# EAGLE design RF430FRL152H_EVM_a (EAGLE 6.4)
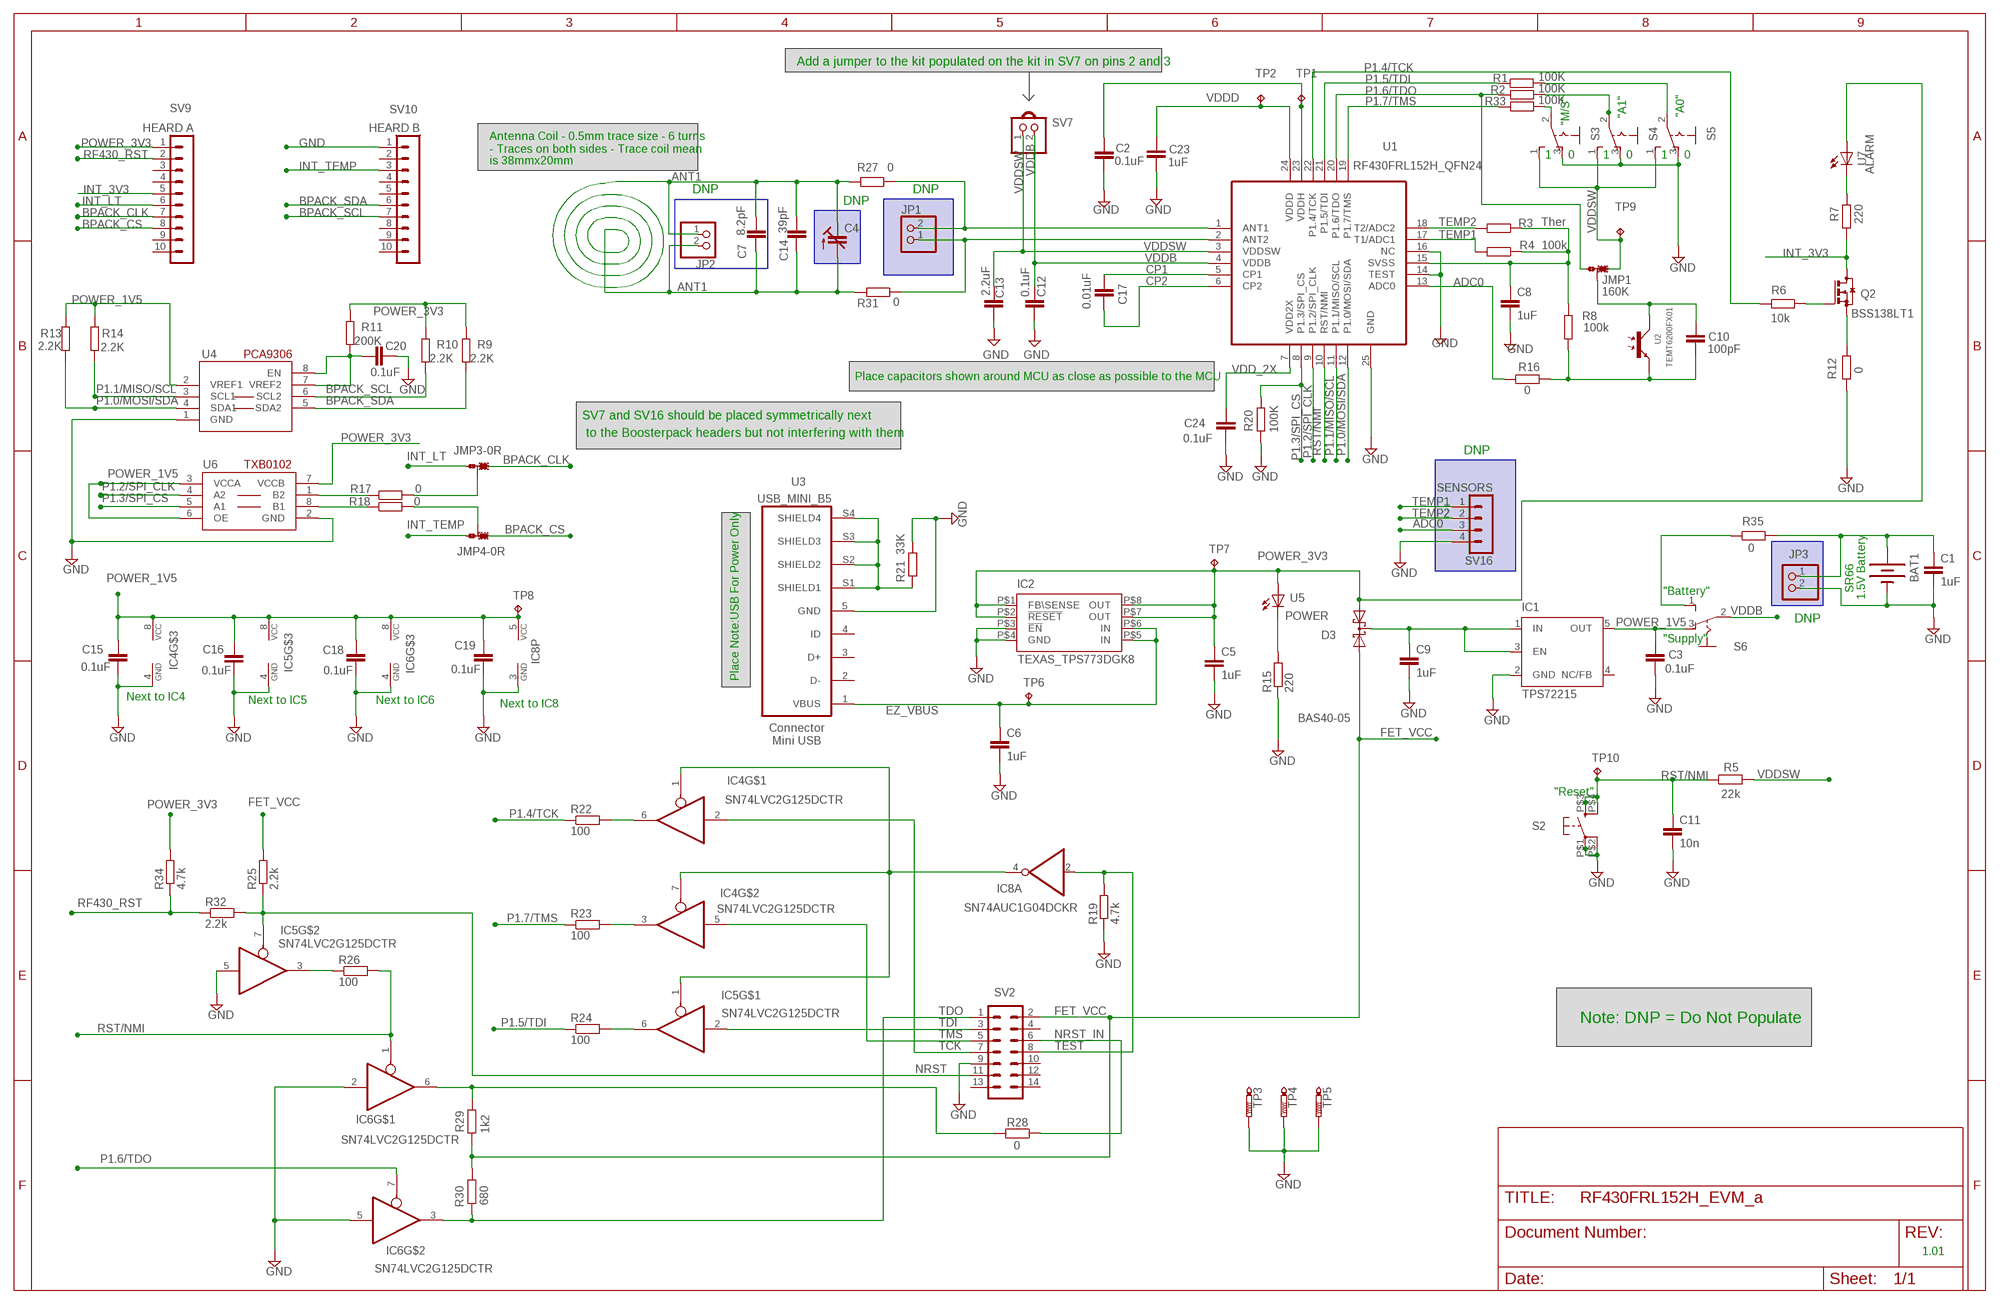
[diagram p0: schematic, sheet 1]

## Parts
BAT1  SPARKFUN_BATTERY12MM  [SPARKFUN_BATTCON_12MM]
C1  1uF  LAUNCHPAD_CAP0603  [ROY_CAP_0603]
C2  0.1uF  LAUNCHPAD_CAP0603  [ROY_CAP_0603]
C3  0.1uF  LAUNCHPAD_CAP0603  [ROY_CAP_0603]
C4  C-TRIMM_C-TRIMM3008  [C-TRIMM_3008]
C5  1uF  LAUNCHPAD_CAP0603  [ROY_CAP_0603]
C6  1uF  LAUNCHPAD_CAP0603  [ROY_CAP_0603]
C7  8.2pF  LAUNCHPAD_CAP0603  [ROY_CAP_0603]
C8  1uF  LAUNCHPAD_CAP0603  [ROY_CAP_0603]
C9  1uF  LAUNCHPAD_CAP0603  [ROY_CAP_0603]
C10  100pF  LAUNCHPAD_CAP0603  [ROY_CAP_0603]
C11  10n  LAUNCHPAD_CAP0603  [ROY_CAP_0603]
C12  0.1uF  LAUNCHPAD_CAP0603  [ROY_CAP_0603]
C13  2.2uF  LAUNCHPAD_CAP0603  [ROY_CAP_0603]
C14  39pF  LAUNCHPAD_CAP0603  [ROY_CAP_0603]
C15  0.1uF  LAUNCHPAD_CAP0603  [ROY_CAP_0603]
C16  0.1uF  LAUNCHPAD_CAP0603  [ROY_CAP_0603]
C17  0.01uF  LAUNCHPAD_CAP0603  [ROY_CAP_0603]
C18  0.1uF  LAUNCHPAD_CAP0603  [ROY_CAP_0603]
C19  0.1uF  LAUNCHPAD_CAP0603  [ROY_CAP_0603]
C20  0.1uF  LAUNCHPAD_CAP0603  [ROY_CAP_0603]
C23  1uF  LAUNCHPAD_CAP0603  [ROY_CAP_0603]
C24  0.1uF  LAUNCHPAD_CAP0603  [ROY_CAP_0603]
D3  BAS40-05  [SOT23]
IC1  TPS72215  TEXAS_TPS77015  [TEXAS_SOT23-DBV]
IC2  TEXAS_TPS773DGK8  [DGK]
IC4  SN74LVC2G125DCTR  APOLLO_74LVC2G125DCT  [APOLLO_SSOP08]
IC5  SN74LVC2G125DCTR  APOLLO_74LVC2G125DCT  [APOLLO_SSOP08]
IC6  SN74LVC2G125DCTR  APOLLO_74LVC2G125DCT  [APOLLO_SSOP08]
IC8  SN74AUC1G04DCKR  74XX-LITTLE-DE_74AUC1G04DCK  [74XX-LITTLE-DE_SC70-5]
JMP1  160K-JUMPB  0R-JUMPB  [B0R-JMP]
JMP3  0R-JUMPB  [B0R-JMP]
JMP4  0R-JUMPB  [B0R-JMP]
JP1  APOLLO_PINHD-1X2  [APOLLO_1X02]
JP2  APOLLO_PINHD-1X2  [APOLLO_1X02]
JP3  APOLLO_PINHD-1X2  [APOLLO_1X02]
Q2  BSS138LT1  BSS123  [SOT23]
R1  100K  LAUNCHPAD_RES0603  [ROY_RES_0603]
R2  100K  LAUNCHPAD_RES0603  [ROY_RES_0603]
R3  Ther  LAUNCHPAD_RES0603  [ROY_RES_0603]
R4  100k  LAUNCHPAD_RES0603  [ROY_RES_0603]
R5  22k  LAUNCHPAD_RES0603  [ROY_RES_0603]
R6  10k  LAUNCHPAD_RES0603  [ROY_RES_0603]
R7  220  LAUNCHPAD_RES0603  [ROY_RES_0603]
R8  100k  LAUNCHPAD_RES0603  [ROY_RES_0603]
R9  2.2K  LAUNCHPAD_RES0603  [ROY_RES_0603]
R10  2.2K  LAUNCHPAD_RES0603  [ROY_RES_0603]
R11  200K  LAUNCHPAD_RES0603  [ROY_RES_0603]
R12  0  LAUNCHPAD_RES0603  [ROY_RES_0603]
R13  2.2K  LAUNCHPAD_RES0603  [ROY_RES_0603]
R14  2.2K  LAUNCHPAD_RES0603  [ROY_RES_0603]
R15  220  LAUNCHPAD_RES0603  [ROY_RES_0603]
R16  0  LAUNCHPAD_RES0603  [ROY_RES_0603]
R17  0  LAUNCHPAD_RES0603  [ROY_RES_0603]
R18  0  LAUNCHPAD_RES0603  [ROY_RES_0603]
R19  4.7k  LAUNCHPAD_RES0603  [ROY_RES_0603]
R20  100K  LAUNCHPAD_RES0603  [ROY_RES_0603]
R21  33K  LAUNCHPAD_RES0603  [ROY_RES_0603]
R22  100  LAUNCHPAD_RES0603  [ROY_RES_0603]
R23  100  LAUNCHPAD_RES0603  [ROY_RES_0603]
R24  100  LAUNCHPAD_RES0603  [ROY_RES_0603]
R25  2.2k  LAUNCHPAD_RES0603  [ROY_RES_0603]
R26  100  LAUNCHPAD_RES0603  [ROY_RES_0603]
R27  0  LAUNCHPAD_RES0603  [ROY_RES_0603]
R28  0  LAUNCHPAD_RES0603  [ROY_RES_0603]
R29  1k2  LAUNCHPAD_RES0603  [ROY_RES_0603]
R30  680  LAUNCHPAD_RES0603  [ROY_RES_0603]
R31  0  LAUNCHPAD_RES0603  [ROY_RES_0603]
R32  2.2k  LAUNCHPAD_RES0603  [ROY_RES_0603]
R33  100K  LAUNCHPAD_RES0603  [ROY_RES_0603]
R34  4.7k  LAUNCHPAD_RES0603  [ROY_RES_0603]
R35  0  LAUNCHPAD_RES0603  [ROY_RES_0603]
S2  HERCULES_LAUNCHPAD_V1.1_LAUNCHPAD_T062ST06B-025FWT01B  [SW-6.1*3.7]
S3  M251  [M251]
S4  M251  [M251]
S5  M251  [M251]
S6  M251  [M251]
SV2  ML14  [ML14]
SV7  APOLLO_PINHD-1X2  [APOLLO_1X02]
SV9  HEARD A  CON-LSTB_MA10-1W  [CON-LSTB_MA10-1W]
SV10  HEARD B  CON-LSTB_MA10-1W  [CON-LSTB_MA10-1W]
SV16  SENSORS  MA04-1  [MA04-1]
TP1  TPB1,27  [B1,27]
TP2  TPB1,27  [B1,27]
TP3  PTR1PAD1-13  [P1-13]
TP4  PTR1PAD1-13  [P1-13]
TP5  PTR1PAD1-13  [P1-13]
TP6  TPB1,27  [B1,27]
TP7  TPB1,27  [B1,27]
TP8  TPB1,27  [B1,27]
TP9  TPB1,27  [B1,27]
TP10  TPB1,27  [B1,27]
U1  RF430FRL152H_QFN24  APOLLO_APOLLO_24PINQFN24  [QFN24]
U2  TEMT6200FX01  LAUNCHPAD_TEMT60006200  [LAUNCHPAD_0805]
U3  USB_MINI_B5  [USB_MINI_B]
U4  SPARKFUN_PCA9306DCU  [MY_DCU_R-PDSO-G8]
U5  POWER  LEDCHIP-LED0603  [CHIP-LED0603]
U6  TXB0102  [DCU_R-PDSO-G8]
U7  ALARM  LEDCHIP-LED0603  [CHIP-LED0603]
U$1  ROY_JUMPER  [ROY_JUMPER]

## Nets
ADC0: R16.1 SV16.3 U1.13(ADC0)
ANT1: C4.+(E) C4.-(A) C7.1 C7.2 C14.1 C14.2 JP2.1 JP2.2 R27.2 R31.2
BPACK_CLK: JMP3.1 SV9.7
BPACK_CLK_N: JMP3.2 R17.2
BPACK_CS: JMP4.3 SV9.8
BPACK_CS_N: JMP4.2 R18.2
BPACK_SCL: R10.2 SV10.7 U4.6(SCL2)
BPACK_SDA: R9.2 SV10.6 U4.5(SDA2)
CP1: C17.2 U1.5(CP1)
CP2: C17.1 U1.6(CP2)
EZ_VBUS: C6.1 IC2.P$5(IN) IC2.P$6(IN) TP6.TP U3.1(VBUS)
FET_VCC: D3.2(A2) R25.2 R29.1 R30.1 SV2.2
GND: BAT1.GND(-) C1.2 C2.2 C3.1 C5.2 C6.2 C8.2 C9.2 C11.2 C12.1 C13.1 C15.1 C16.1 C18.1 C19.1 C20.1 C23.2 C24.1 IC1.2(GND) IC2.P$3(!EN) IC2.P$4(GND) IC4.4(GND) IC5.4(GND) IC5.5(I) IC6.2(I) IC6.4(GND) IC6.5(I) IC8.3(P:GND) JP3.2 R12.1 R15.1 R19.1 R20.1 R21.2 S2.P$1 S2.P$2 S3.3(S) S4.3(S) S5.3(S) SV2.9 SV10.1 SV16.4 TP3.TP TP4.TP TP5.TP U1.14(TEST) U1.16(NC) U1.25(GND) U3.5(GND) U4.1(GND) U6.2(GND)
INT_3V3: Q2.3(D) R7.1 SV9.5
INT_LT: JMP3.3 SV9.6
INT_TEMP: JMP4.1 SV10.3
N$1: C9.1 D3.3(C) IC1.1(IN) IC1.3(EN)
N$2: C10.1 R8.2 R16.2 U2.2(E)
N$4: JP1.2 R27.1 U1.1(ANT1)
N$5: C8.1 R3.1 R4.1 R8.1 U1.15(SVSS)
N$6: JP1.1 R31.1 U1.2(ANT2)
N$7: R7.2 U7.C
N$8: R35.1 S6.1(O)
N$9: C20.2 R11.2 U4.7(VREF2) U4.8(EN)
N$10: R15.2 U5.C
N$12: Q2.2(S) R12.2
N$13: Q2.1(G) R6.1
N$14: BAT1.PWR@1(+) C1.1 JP3.1 R35.2
N$15: R1.2 S5.2(P)
N$17: R17.1 U6.1(B2)
N$18: R18.1 U6.8(B1)
N$21: C10.2 JMP1.2 U2.1(C)
N$22: R21.1 U3.S1(SHIELD1) U3.S2(SHIELD2) U3.S3(SHIELD3) U3.S4(SHIELD4)
N$23: IC4.1(OE) IC4.7(OE) IC5.1(OE) IC8.4(A:O)
N$24: IC4.6(O) R22.2
N$25: IC4.3(O) R23.2
N$26: IC5.6(O) R24.2
N$27: R2.1 S4.2(P)
N$28: IC5.3(O) R26.1
N$29: R33.1 S3.2(P)
N$30: IC6.6(O) R28.2 R29.2
NRST: IC5.7(OE) R25.1 R32.2 SV2.11
NRST_IN: R28.1 SV2.6
P1.0/MOSI/SDA: R13.2 U1.12(P1.0/MOSI/SDA) U4.4(SDA1)
P1.1/MISO/SCL: R14.2 U1.11(P1.1/MISO/SCL) U4.3(SCL1)
P1.2/SPI_CLK: U1.9(P1.2/SPI_CLK) U6.4(A2)
P1.3/SPI_CS: R20.2 U1.8(P1.3/SPI_CS) U6.5(A1)
P1.4/TCK: R6.2 R22.1 U1.22(P1.4/TCK)
P1.5/TDI: R1.1 R24.1 U1.21(P1.5/TDI)
P1.6/TDO: IC6.7(OE) JMP1.3 R2.2 U1.20(P1.6/TDO)
P1.7/TMS: R23.1 R33.2 U1.19(P1.7/TMS)
POWER_1V5: C3.2 C15.2 C16.2 C18.2 C19.2 IC1.5(OUT) IC4.8(VCC) IC5.8(VCC) IC6.8(VCC) IC8.5(P:VCC) R13.1 R14.1 S6.3(S) TP8.TP U4.2(VREF1) U6.3(VCCA) U6.6(OE)
POWER_3V3: C5.1 D3.1(A1) IC2.P$1(FB\SENSE) IC2.P$2(!RESET) IC2.P$7(OUT) IC2.P$8(OUT) R9.1 R10.1 R11.1 R34.2 SV9.1 TP7.TP U5.A U6.7(VCCB) U7.A
RF430_RST: R32.1 R34.1 SV9.2
RST/NMI: C11.1 IC6.1(OE) R5.1 R26.2 S2.P$3 S2.P$4 TP10.TP U1.10(RST/NMI)
TCK: IC4.2(I) SV2.7
TDI: IC5.2(I) SV2.3
TDO: IC6.3(O) R30.2 SV2.1
TEMP1: R4.2 SV16.1 U1.17(T1/ADC1)
TEMP2: R3.2 SV16.2 U1.18(T2/ADC2)
TEST: IC8.2(A:I) R19.2 SV2.8
TMS: IC4.5(I) SV2.5
VDD_2X: C24.2 U1.7(VDD2X)
VDDB: C12.2 S6.2(P) SV7.2 U1.4(VDDB)
VDDD: C23.1 TP2.TP U1.24(VDDD)
VDDH: C2.1 TP1.TP U1.23(VDDH)
VDDSW: C13.2 JMP1.1 R5.2 S3.1(O) S4.1(O) S5.1(O) SV7.1 TP9.TP U1.3(VDDSW)
Unconnected: IC1.4(NC/FB) SV2.4 SV2.10 SV2.12 SV2.13 SV2.14 SV9.3 SV9.4 SV9.9 SV9.10 SV10.2 SV10.4 SV10.5 SV10.8 SV10.9 SV10.10 U3.2(D-) U3.3(D+)

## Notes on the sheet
- Add a jumper to the kit populated on the kit in SV7 on pins 2 and 3
- "M/S" | "A1" | "A0"
- Pickup coil
- Antenna Coil - 0.5mm trace size - 6 turns
- - Traces on both sides - Trace coil mean
- 1 | 0 | 1 | 0 | 1 | 0
- is 38mmx20mm
- DNP | DNP
- DNP
- JMP1
- 160K
- Place capacitors shown around MCU as close as possible to the MCU
- SV7 and SV16 should be placed symmetrically next
- to the Boosterpack headers but not interfering with them
- DNP
- "Battery" | SR66
- 1.5V Battery
- DNP
- "Supply"
- Place Note:USB For Power Only
- Next to IC4
- Next to IC5 | Next to IC6
- Next to IC8
- Connector
- Mini USB
- "Reset"
- Note: DNP = Do Not Populate
- 1.01

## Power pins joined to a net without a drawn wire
ID: U3.4(ID)

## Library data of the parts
BAT1 = RF430FRL152H_EVM_a:SPARKFUN_BATTERY: Battery Holders
C1-C3 C5-C20 C23 C24 = roy:LAUNCHPAD_CAP
C4 = RF430FRL152H_EVM:C-TRIMM_C-TRIMM: Trimm capacitor; OC_FARNELL: unknown; OC_NEWARK: unknown
D3 = diode:BAS40-05: Silicon Schottky Diodes General-purpose diode for high-speed switching
IC1 = RF430FRL152H_EVM_a:TEXAS_TPS770*: ULTRALOW-POWER 50-mA LOW-DROPOUT LINEAR REGULATORS 50-mA Low-Dropout Regulator Source: http://focus.ti.com/lit/ds/symlink/tps77001.pdf; MF: TEXAS INSTRUMENT CONNECTORS; MPN: TPS77015DBVT; OC_FARNELL: 1412879; OC_NEWARK: 77C1175
IC2 = RF430FRL152H_EVM_a:TEXAS_TPS773*: 250-mA LDO REGULATORS WITH RESET OUTPUT WITH 8-PIN MSOP PACKAGING Source: http://focus.ti.com/lit/ds/symlink/tps77333.pdf
IC4-IC6 = RF430FRL152H_EVM_a:APOLLO_74*2G125: Dual line drivers with 3-state outputs.
IC8 = RF430FRL152H_EVM_a:74XX-LITTLE-DE_74*1G04: INVERTER Gate
JMP1 JMP3 JMP4 = jump-0r-smd:0R-JUMP: SMD 0R 0805 Jumper
JP1-JP3 SV7 = RF430FRL152H_EVM:APOLLO_PINHD-1X2: PIN HEADER
Q2 = transistor-small-signal:BSS123: N-CHANNEL MOS FET
R1-R35 = roy:LAUNCHPAD_RES
S2 = yw8:HERCULES_LAUNCHPAD_V1.1_LAUNCHPAD_T062S
S3-S6 = switch:M251: SLIDING SWITCH Mors, distributor Buerklin, 11G702
SV2 = con-ml:ML14: HARTING; OC_FARNELL: unknown; OC_NEWARK: unknown
SV9 SV10 = RF430FRL152H_EVM_a:CON-LSTB_MA10-1W: PIN HEADER; OC_FARNELL: unknown; OC_NEWARK: unknown
SV16 = con-lstb:MA04-1: PIN HEADER; OC_FARNELL: unknown; OC_NEWARK: unknown
TP1 TP2 TP6-TP10 = testpad:TP: Test pad
TP3-TP5 = testpad:PTR1: TEST PIN
U1 = RF430FRL152H_EVM_a:APOLLO_APOLLO_24PIN
U2 = roy:LAUNCHPAD_TEMT6000
U3 = susbfet:USB_MINI_B5
U4 = RF430FRL152H_EVM_a:SPARKFUN_PCA9306
U5 U7 = led:LED: LED
U6 = My:TXB0102
U$1 = roy:ROY_JUMPER

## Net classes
1 Ground: width 0.203 mm, drill 0.61 mm

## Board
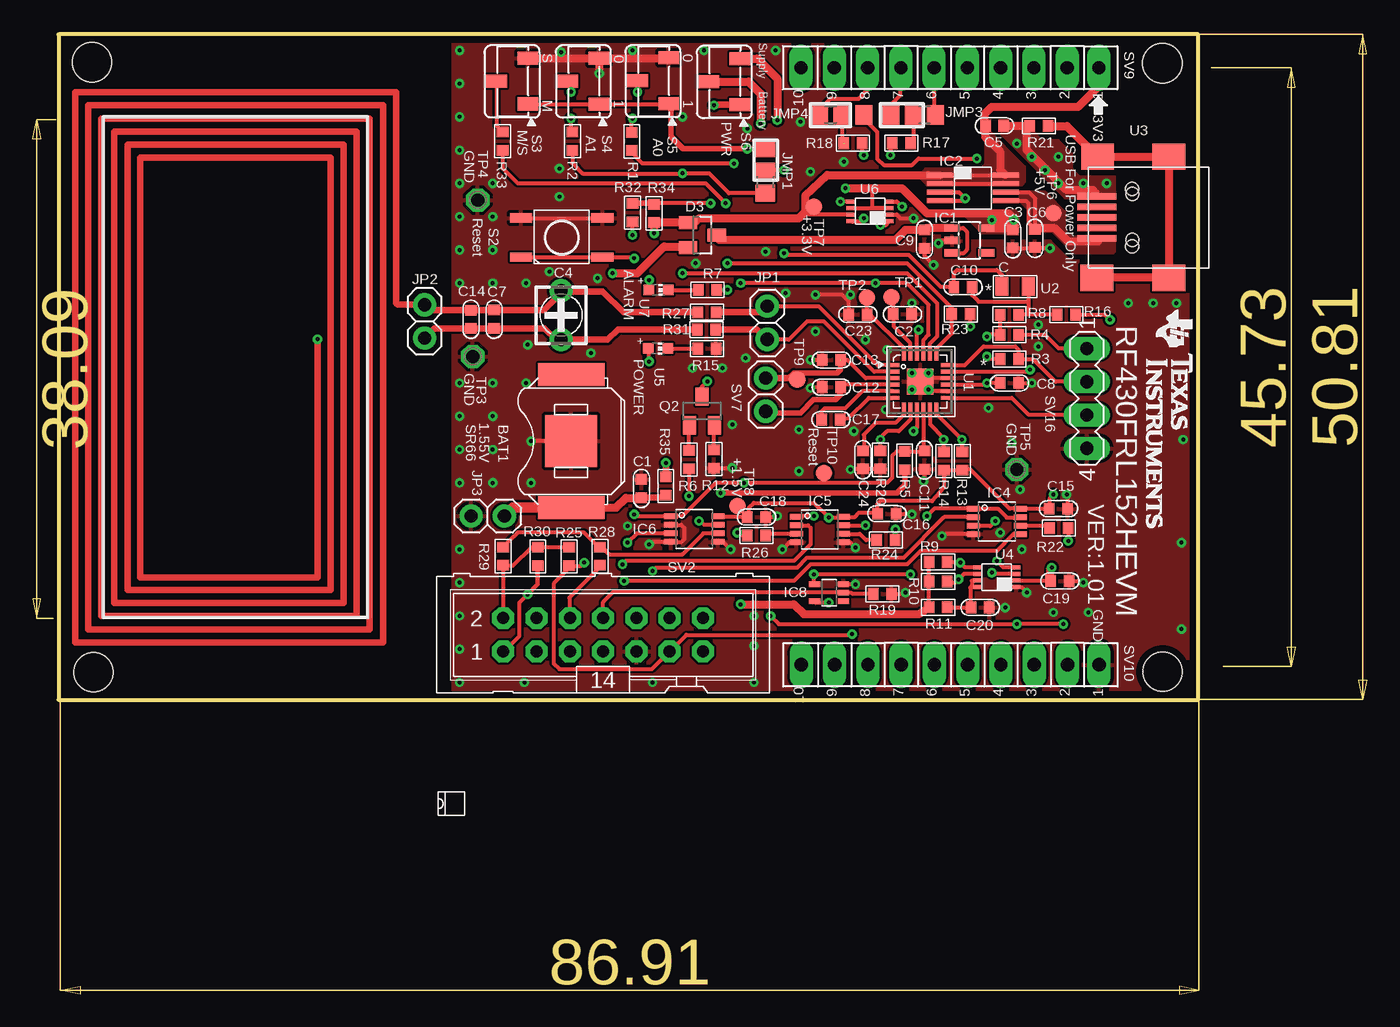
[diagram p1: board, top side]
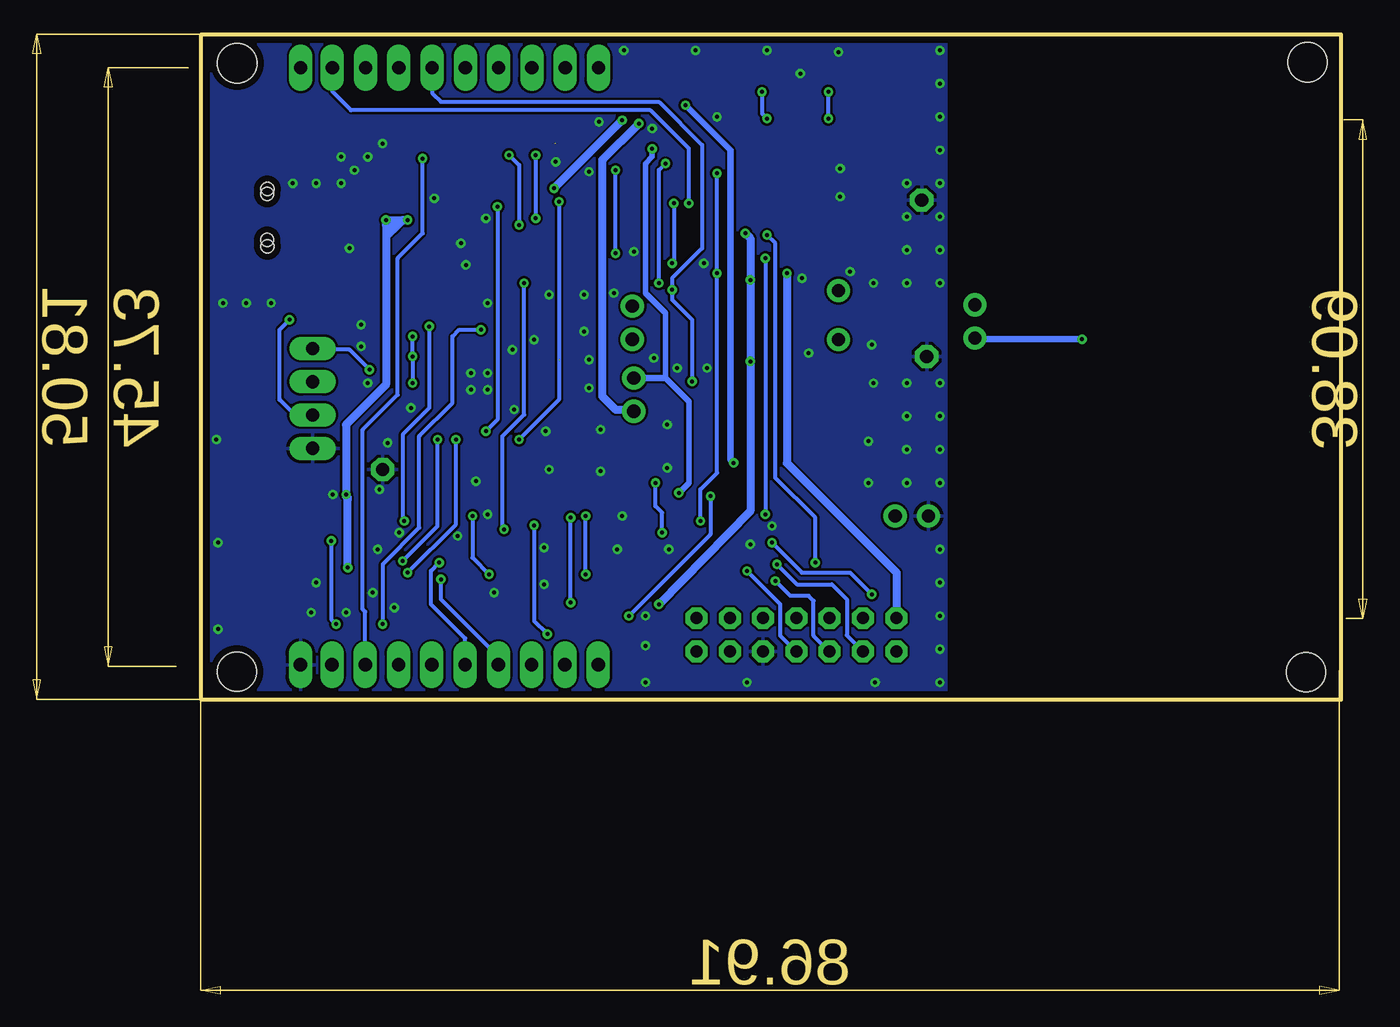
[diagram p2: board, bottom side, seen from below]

Size 101.84 x 73.3 mm. Coordinates in mm from the lower left corner, seen from the top.
Outline: 1.98,22.47 88.98,22.47 88.98,73.28 1.98,73.28 1.98,22.47
Copper layers (1*16): Top 0.035mm / dielectric 1.5mm / Bottom 0.035mm
Design rules "default": minimum track width 8mil, minimum drill 10mil, track to track 7mil, track to pad 7mil, pad to pad 7mil, via to via 7mil, smd to smd 0mil, copper to edge 20mil, drill to drill 10mil, minimum pad ring 15mil, minimum via ring 8mil, stop-mask expansion 4mil, vias tented up to drill 0mil, thermal gap 10mil
Holes 3 mm at 4.52,71.15 4.65,24.57 86.25,24.61 86.24,71.07
Holes 1 mm at 83.95,61.09 83.95,57.58

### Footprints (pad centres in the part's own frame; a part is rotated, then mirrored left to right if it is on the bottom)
SPARKFUN_BATTCON_12MM = smd 3.962 x 3.962: GND 0,0 | smd 1.778 x 5.08: PWR@1 -5.08,0; PWR@2 5.08,0
ROY_CAP_0603 = smd 0.8 x 0.9: 1 -0.7,0; 2 0.7,0
C-TRIMM_3008 = drill 1: + -1.875,0; - 1.875,0
SOT23 = smd 1 x 1.4: 1 -0.95,-1.1; 2 0.95,-1.1; 3 0,1.1
TEXAS_SOT23-DBV = smd 0.55 x 1.2: 1 -0.95,-1.3; 2 0,-1.3; 3 0.95,-1.3; 4 0.95,1.3; 5 -0.95,1.3
DGK = smd 0.4 x 2: P$1 0,0; P$2 0.65,0; P$3 1.3,0; P$4 1.95,0; P$5 1.95,5.05; P$6 1.3,5.05; P$7 0.65,5.05; P$8 0,5.05
APOLLO_SSOP08 = smd 0.4 x 1: 1 -0.975,-1.8; 2 -0.325,-1.8; 3 0.325,-1.8; 4 0.975,-1.8; 5 0.975,1.8; 6 0.325,1.8; 7 -0.325,1.8; 8 -0.975,1.8
74XX-LITTLE-DE_SC70-5 = smd 0.4 x 0.85: 1 -0.65,-1.1; 2 0,-1.1; 3 0.65,-1.1; 4 0.65,1.1; 5 -0.65,1.1
B0R-JMP = smd 1.5 x 1.3: 1 0,1.7; 2 0,0; 3 0,-1.7
APOLLO_1X02 = drill 1.016: 1 -1.27,0; 2 1.27,0
ROY_RES_0603 = smd 0.8 x 0.9: 1 -0.7,0; 2 0.7,0
SW-6.1*3.7 = smd 1.7 x 0.7: P$1 -3.1,1.5; P$2 3.1,1.5; P$3 -3.1,-1.5; P$4 3.1,-1.5
M251 = smd 1 x 1.6: 1 -1.75,-1.2; 2 0,1.2; 3 1.75,-1.2
ML14 = drill 0.914 octagon: 1 -7.62,-1.27; 2 -7.62,1.27; 3 -5.08,-1.27; 4 -5.08,1.27; 5 -2.54,-1.27; 6 -2.54,1.27; 7 0,-1.27; 8 0,1.27; 9 2.54,-1.27; 10 2.54,1.27; 11 5.08,-1.27; 12 5.08,1.27; 13 7.62,-1.27; 14 7.62,1.27
CON-LSTB_MA10-1W = drill 1.016 long: 1 -11.303,0; 2 -8.89,0; 3 -6.35,0; 4 -3.81,0; 5 -1.27,0; 6 1.27,0; 7 3.81,0; 8 6.35,0; 9 8.89,0; 10 11.43,0
MA04-1 = drill 1.016 long: 1 -3.81,0; 2 -1.27,0; 3 1.27,0; 4 3.81,0
B1,27 = smd 1.27 x 1.27: TP 0,0
P1-13 = drill 1 pad 1.676 octagon: TP 0,0
QFN24 = smd 1 x 0.3: 1 -2.1,1.25; 2 -2.1,0.75; 3 -2.1,0.25; 4 -2.1,-0.25; 5 -2.1,-0.75; 6 -2.1,-1.25; 13 2.1,-1.25; 14 2.1,-0.75; 15 2.1,-0.25; 16 2.1,0.25; 17 2.1,0.75; 18 2.1,1.25 | smd 0.3 x 1: 7 -1.25,-2.1; 8 -0.75,-2.1; 9 -0.25,-2.1; 10 0.25,-2.1; 11 0.75,-2.1; 12 1.25,-2.1; 19 1.25,2.1; 20 0.75,2.1; 21 0.25,2.1; 22 -0.25,2.1; 23 -0.75,2.1; 24 -1.25,2.1 | smd 2 x 2: 25 0,0
LAUNCHPAD_0805 = smd 1 x 1.4: 1 -1,0; 2 1,0
USB_MINI_B = smd 0.5 x 3: 1 -1.6,8.55; 2 -0.8,8.55; 3 0,8.55; 4 0.8,8.55; 5 1.6,8.55 | smd 2 x 2.5: S1 -4.6,8.55; S2 -4.6,3.05; S3 4.65,3.05; S4 4.65,8.5 | hole 1.016: -2.2,5.85; 2.2,5.85
MY_DCU_R-PDSO-G8 = smd 0.3 x 0.6: 1 -0.75,-1.5; 2 -0.25,-1.5; 3 0.25,-1.5; 4 0.75,-1.5; 5 0.75,1.5; 6 0.25,1.5; 7 -0.25,1.5; 8 -0.75,1.5
CHIP-LED0603 = smd 0.8 x 0.8: A 0,-0.75; C 0,0.75
DCU_R-PDSO-G8 = smd 0.3 x 0.6: 1 -0.75,-1.5; 2 -0.25,-1.5; 3 0.25,-1.5; 4 0.75,-1.5; 5 0.75,1.5; 6 0.25,1.5; 7 -0.25,1.5; 8 -0.75,1.5

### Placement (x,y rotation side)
BAT1  41.1,42.22 90 top
C1  46.46,38.6 90 top
C2  66.4,51.91 0 top
C3  74.81,57.66 90 top
C4  40.33,51.83 270 top
C5  73.43,66.31 0 top
C6  76.5,57.7 270 top
C7  35.22,51.52 90 top
C8  74.56,46.67 0 top
C9  68.09,57.63 270 top
C10  71.02,53.98 180 top
C11  68.09,40.77 270 top
C12  60.97,46.34 0 top
C13  60.97,48.42 0 top
C14  33.45,51.52 90 top
C15  78.31,37.05 180 top
C16  65.22,36.67 180 top
C17  60.94,43.86 180 top
C18  55.26,36.41 180 top
C19  78.42,31.53 180 top
C20  72.33,29.51 180 top
C23  62.99,51.89 180 top
C24  63.37,40.79 90 top
D3  51.12,57.95 270 top
IC1  71.5,57.54 270 top
IC2  69.25,62.52 270 top
IC4  73.61,36.08 270 top
IC5  60.09,35.46 270 top
IC6  50.51,35.5 270 top
IC8  60.8,30.65 90 top
JMP1  55.93,62.83 0 top
JMP3  67.23,67.12 90 top
JMP4  61.76,67.13 270 top
JP1  56.07,51.25 90 top
JP2  29.91,51.35 270 top
JP3  34.74,36.5 180 top
Q2  51.09,44.52 0 top
R1  45.73,65.1 90 top
R2  41.2,65.12 270 top
R3  74.56,48.49 0 top
R4  74.55,50.34 0 top
R5  66.57,40.73 270 top
R6  50.11,40.8 270 top
R7  51.51,53.76 180 top
R8  74.55,51.86 0 top
R9  69.13,32.99 0 top
R10  69.13,31.51 0 top
R11  69.13,29.53 0 top
R12  52,40.85 90 top
R13  70.97,40.69 90 top
R14  69.57,40.69 90 top
R15  51.48,49.29 180 top
R16  78.91,51.88 180 top
R17  66.31,64.96 0 top
R18  62.62,64.97 180 top
R19  64.87,30.55 180 top
R20  64.72,40.8 90 top
R21  76.8,66.28 180 top
R22  78.35,35.57 180 top
R23  70.86,51.91 0 top
R24  65.13,34.67 180 top
R25  40.94,33.4 90 top
R26  55.25,35.02 180 top
R27  51.48,52.06 180 top
R28  43.3,33.43 90 top
R29  35.9,33.43 90 top
R30  38.56,33.41 270 top
R31  51.43,50.74 180 top
R32  45.78,59.67 270 top
R33  35.87,65.12 270 top
R34  47.44,59.61 270 top
R35  48.33,38.78 270 top
S2  40.38,57.76 0 top
S3  36.6,69.71 90 top
S4  42.04,69.71 90 top
S5  47.35,69.73 90 top
S6  52.79,69.67 90 top
SV2  43.54,27.43 0 top
SV7  55.95,45.77 270 top
SV9  70.08,70.73 180 top
SV10  70.1,25.14 180 top
SV16  80.48,45.48 270 top
TP1  65.55,53.22 0 top
TP2  63.68,53.19 0 top
TP3  33.6,48.69 0 top
TP4  33.98,60.62 0 top
TP5  75.13,40.05 0 top
TP6  77.92,59.61 0 top
TP7  59.63,60.12 0 top
TP8  53.79,37.26 0 top
TP9  58.36,46.91 0 top
TP10  60.39,39.8 0 top
U1  67.75,46.77 0 top
U2  75,54.02 0 top
U3  89.79,59.29 90 top
U4  73.6,31.82 90 top
U5  47.74,49.29 270 top
U6  63.92,59.77 90 top
U7  47.78,53.76 270 top
U$1  32.99,13.65 90 top
U$4  [LOGO16_TPLACE]  84.83,52.34 270 top

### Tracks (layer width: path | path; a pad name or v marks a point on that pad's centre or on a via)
ADC0  (via drill 0.3)
  Top 0.305: SV16.3 76.05,44.21 74.73,45.52 U1.13 | R16.1 81.84,51.88 v82.24,51.48
  Bottom 0.305: SV16.3 81.82,44.21 83,45.39 83,50.72 v82.24,51.48
ANT1  (via drill 0.3)
  Top 0.5: v21.73,50 21.73,31.82 8.21,31.82 8.21,63.85 22.73,63.85 22.73,30.85 7.23,30.85 7.23,64.85 23.73,64.85 23.73,29.85 6.23,29.85 6.23,65.85 24.73,65.85 24.73,28.85 5.23,28.85 5.23,66.85 25.73,66.85 25.73,27.85 4.23,27.85 4.23,67.85 26.73,67.85 26.73,26.85 3.23,26.85 3.23,68.85 27.73,68.85 27.73,52.77 27.88,52.62 JP2.1 30.45,52.22 C14.2 38.39,52.22 C7.2 39.04,52.22 40.46,53.64 41.41,53.64 C4.+ 41.54,53.64 43.5,53.64 45.09,52.06 R27.2 | JP2.2 30.65,50.82 C14.1 38.39,50.82 C7.1 39.08,50.82 39.95,49.96 41.48,49.96 C4.- 43.88,49.95 44.67,50.74 R31.2
  Bottom 0.5: v21.73,50 29.49,50 JP2.2
BPACK_CLK
  Top 0.305: JMP3.1 65.53,67.92 66.24,68.63 66.24,70.66 | 66.24,70.66 66.24,70.78 | SV9.7 66.27,70.7 66.24,70.66
BPACK_CLK_N
  Top 0.305: JMP3.2 67.23,65.18 R17.2
BPACK_CS
  Top 0.305: JMP4.3 60.06,67.53 60.9,68.37 63.06,68.37 63.7,69.01 63.7,70.69 SV9.8
BPACK_CS_N  (1 unrouted)
  Top 0.305: JMP4.2 61.76,65.1 61.92,64.94
BPACK_SCL  (via drill 0.3)
  Top 0.305: R10.2 70.01,31.38 70.4,31.38 v70.68,31.67 71.06,32.05 71.06,32.07 U4.6
  Bottom 0.305: SV10.7 66.29,25.76 70.68,30.14 v70.68,31.67
BPACK_SDA  (via drill 0.3)
  Top 0.305: U4.5 71.17,32.57 v70.81,32.94 70.38,32.94 R9.2
  Bottom 0.305: SV10.6 68.83,27.16 71.44,29.76 71.44,32.3 v70.81,32.94
CP1
  Top 0.305: U1.5 63.33,46.02 62.02,44.72 60.45,44.72 60.23,44.49 60.23,43.99 C17.2
CP2
  Top 0.305: C17.1 62.29,43.98 63.83,45.52 U1.6 | U1.6
EZ_VBUS
  Top 0.305: 76.59,58.4 76.58,58.4 C6.1 76.01,58.89 76.01,60.37 75.82,60.57 IC2.P$5 | IC2.P$6 76.06,61.22 76.52,60.75 76.52,58.34
  Top 0.406: U3.1 81.37,57.47 81.35,57.45
  Top 0.61: 81.35,57.45 79.06,57.45 78.05,58.47 76.65,58.47 76.59,58.4 76.4,58.47
  pour Top (no thermals): 76.14,61.26 77.28,61.26 77.41,61.13 78.81,59.74 78.81,58.34 79.32,57.83 82.62,57.83 82.62,56.69 82.49,56.56 79.44,56.56 77.79,58.21 76.65,58.21 76.01,58.85 76.01,59.86 75.38,60.5 75.38,61.26
FET_VCC  (via drill 0.3)
  Top 0.305: SV2.2 35.9,28.72 R29.1 35.94,32.69 36.65,32.69 38.07,34.11 R30.1 38.57,34.1 | R25.2 38.57,34.1 | 38.57,34.1 38.55,34.08
  Top 0.61: v44.26,55.04 46.17,55.04 48.2,57.07 49.96,57.07 D3.2
  Bottom 0.61: v44.26,55.04 44.26,40.54 35.9,32.18 35.9,28.72 SV2.2
GND  (via drill 0.3)
  Top 0.305: C8.2 76.26,46.67 v76.27,46.66 | IC4.4 69.68,35.11 v69.41,34.97 | U4.1 75.47,31.07 v75.89,30.65 | C16.1 66.57,36.67 v67.12,36.62 | C15.1 79.01,38.08 v78.94,38.15 | IC5.5 62.4,34.49 v62.81,34.08 | IC6.5 52.71,34.53 v53.28,33.95 | C18.1 56.75,36.41 v56.84,36.5 | IC5.4 57.75,34.49 v57.22,33.95 | C3.1 76.46,56.96 C6.2 77.61,57 v77.67,56.94 | 43.49,71.46 S4.3 | S2.P$1 S2.P$2 | R20.1 63.51,40.1 C24.1 62.46,40.09 v62.43,40.05 | C11.2 68.09,39.23 v68.01,39.16 | R12.1 53.38,40.15 v53.41,40.18 | C19.1 80.09,31.53 v80.21,31.41 | IC8.3 62.67,31.3 v62.81,31.29 | R19.1 66.21,30.55 v66.62,30.65 | v47.06,34.34 47.25,34.53 IC6.4 49.54,34.53 49.73,34.72 49.73,35.61 49.5,35.83 IC6.2 | BAT1.GND 38.31,42.22 v38.04,42.21 | C2.2 67.08,52.29 v67.12,52.75 | U6.2 65.95,59.52 66.24,59.23 v67.25,59.23 | IC2.P$4 71,60.57 v71.19,60.75 70.72,61.22 IC2.P$3 | C9.2 68.09,56.36 v68.78,55.67 | IC1.2 69.37,57.54 v69.16,57.32 | C13.1 v59.39,48.42 v59.38,48.43 | C12.1 60.08,46.34 v59.38,46.27 | C23.2 62.29,52.88 61.79,53.39 v59.76,53.39 | U1.14 68.5,46.02 | 68.5,46.02 U1.25 68,47.02 U1.16 | v68.4,46.15 68.52,46.02 68.5,46.02
  Top 0.406: U3.5 81.24,61.24 80.97,61.39
  Top 0.61: S3.3 43.49,71.46 43.59,71.46 43.63,71.42 | S5.3 48.53,71.46 S4.3 43.24,70.41 v43.25,70.28 | 80.97,61.39 78.93,61.39 77.28,63.05 75.89,64.44 75.89,66.07 R21.2 76.07,66.3 C5.2
  other vias: 78.3,61.89 77.28,62.91 76.27,63.93 75.13,64.94 78.3,63.93 80.21,61.89 81.98,61.89 32.58,72.05 32.58,69.52 32.58,66.97 32.58,64.44 32.58,61.89 32.58,59.36 32.58,56.81 32.58,54.28 32.58,46.66 32.58,44.11 32.58,41.58 32.58,39.03 37.53,23.79 32.58,33.95 32.58,31.41 32.58,28.88 32.58,26.34 32.58,23.79 35.12,46.66 35.12,44.11 35.12,41.58 35.12,39.03 47.31,23.79 35.12,54.28 35.12,56.81 35.12,59.36 35.12,61.89 37.66,54.28 37.66,46.66 49.6,66.97 50.36,47.8 52.65,47.8 42.61,48.94 37.79,49.58 39.44,55.16 43.12,54.66 59.76,50.59 63.57,49.96 65.22,49.19 65.09,44.62 62.68,42.97 58.49,43.1 53.41,43.48 55.06,28.88 55.06,26.59 55.06,23.79 77.92,29.13 74.24,29.51 80.59,29.13 74.75,42.08 75.38,38.53 87.32,52.75 85.54,52.75 83.63,52.75 76.78,51.1 76.78,49.45 56.71,72.05 67.12,47.42 68.4,47.42 67.12,46.15 45.41,35.73 38.04,39.03 62.43,53.39 73.86,35.23 75.51,33.95 55.95,56.69 54.55,66.09 58.62,66.59 61.92,63.55 59.38,62.78 40.2,60.88 40.2,63.04 51.25,72.05 45.79,72.05 40.33,71.93 54.43,48.56 58.49,39.92 72.97,44.75 87.7,27.86 87.7,34.46 87.83,42.34 57.47,53.51 50.62,55.8
  pour Top: 32.07,73.2 32.07,22.52 32.2,22.4 88.97,22.4 88.72,54.78 88.72,55.93 79.19,55.93 77.67,57.45 70.55,57.45 70.43,57.58 67.12,61.39 67,67.36 88.72,67.23 88.72,73.2
  pour Top (no thermals): 81.73,62.4 79.95,62.4 79.32,63.04 79.32,64.18 78.3,65.2 77.03,65.2 76.4,65.83 75.76,66.47 74.11,66.47 73.98,66.34 73.98,65.58 78.81,60.75 82.49,60.75 82.62,60.88 82.62,62.4
  pour Bottom: 32.07,73.2 88.97,73.2 88.97,22.52 32.07,22.52
INT_3V3  (via drill 0.3)
  Top 0.305: R7.1 v53.03,53.76 v53.03,53.77 | Q2.3 51.1,46.38 v51.5,46.78
  Bottom 0.305: v51.5,46.78 51.5,51.48 53.03,53 v53.03,53.77 53.03,54.66 50.74,56.94 50.74,64.82 54.04,68.12 70.68,68.12 71.35,68.79 SV9.5
INT_LT
  Top 0.305: SV9.6 68.81,67.24 JMP3.3
INT_TEMP  (via drill 0.3)
  Top 0.305: JMP4.1 63.46,66.83 64.46,65.83 64.46,63.8 64.97,63.29 67.12,63.29 67.63,63.8 v72.08,63.8
  Bottom 0.305: SV10.3 76.45,29.19 76.65,29.38 76.65,43.1 73.98,45.77 73.98,56.18 72.08,58.08 v72.08,63.8
N$1
  Top 0.305: IC1.1 71.04,58.49 71.32,58.21 71.32,56.81 71.09,56.59 IC1.3
  Top 0.61: IC1.1 68.24,58.49 C9.1 66.61,58.33 65.85,57.58 52.39,57.58 52.27,57.96 D3.3
N$2
  Top 0.305: R16.2 75.89,51.88 | 75.89,51.88 75.63,51.88 | 75.63,51.88 75.28,51.88 75.13,51.73 | R8.2 75.61,51.86 75.63,51.88 | U2.2 76,52.98 | 76,52.98 76,52 75.89,51.88 | C10.1 71.72,53.36 72.23,52.85 75.87,52.85 76,52.98
N$4
  Top 0.305: U1.1 64.49,48.02 60.01,52.5 56.09,52.5 JP1.2
  Top 0.5: R27.1 55.48,52.06 JP1.2
N$5  (via drill 0.3)
  Top 0.305: 73.85,48.62 R3.1 73.04,48.49 v72.84,48.69 | 73.86,46.92 C8.1 72.85,46.67 v72.84,46.66 72.71,46.52 U1.15 | R8.1 R4.1 72.97,50.34 v72.84,50.21
  Bottom 0.305: v72.84,50.21 v72.84,48.69 72.84,47.92 v72.84,46.66
N$6
  Top 0.305: U1.2 64.22,47.52 60.39,51.35 59.12,51.35 57.73,49.96 56.09,49.96 JP1.1
  Top 0.5: R31.1 55.31,50.74 JP1.1
N$7
  Top 0.305: U7.C R7.2
N$8  (via drill 0.3)
  Top 0.5: S6.1 52.06,67.92 v52.01,67.86 | v48.33,40.56 R35.1
  Bottom 0.5: v52.01,67.86 48.58,64.44 48.58,40.81 v48.33,40.56
N$9
  Top 0.305: U4.7 71.73,31.57 71.7,31.54 71.7,31.16 | 71.7,31.16 71.57,31.03 71.57,29.57 C20.2 71.61,29.53 R11.2 | U4.8 71.78,31.07 71.7,31.16
N$10
  Top 0.305: U5.C R15.2
N$12
  Top 0.305: R12.2 52,43.38 Q2.2
N$13
  Top 0.305: R6.1 50.11,43.39 Q2.1
N$14
  Top 0.5: C1.1 48.15,37.9 R35.2
  Top 0.61: BAT1.PWR@1 44.53,37.14 45.28,37.89 C1.1
  Top 0.813: JP3.1 36.66,37.14 BAT1.PWR@1
N$15  (via drill 0.3)
  Top 0.305: S5.2 46.15,68.89 v46.17,68.88 | R1.2 45.73,66.79 v45.79,66.85
  Bottom 0.305: v46.17,68.88 46.17,67.23 46.11,67.17 v45.79,66.85
N$17  (via drill 0.3)
  Top 0.305: R17.1 65.49,64.83 v65.47,64.05 | v64.71,58.72 65.12,58.72 U6.1
  Bottom 0.305: v65.47,64.05 64.71,63.29 v64.71,58.72
N$18  (via drill 0.3)
  Top 0.305: R18.1 63.29,64.33 v63.44,64.05 | v63.44,59.23 63.19,58.97 62.59,58.97 U6.8
  Bottom 0.305: v63.44,64.05 v63.44,59.23
N$21  (via drill 0.3)
  Top 0.305: v57.35,56.56 57.73,56.43 66.87,56.43 69.32,53.98 C10.2 70.32,55.06 70.55,55.29 73.6,55.29 74,54.89 U2.1 | v57.35,62.91 56.36,62.91 JMP1.2
  Bottom 0.305: v57.35,56.56 v57.35,62.91
N$22
  Top 0.61: R21.1 78.95,66.28 U3.S4 U3.S3 U3.S2 U3.S1
N$23  (via drill 0.3)
  Top 0.305: IC4.7 75.37,36.37 74.36,36.37 73.67,37.06 IC4.1 68.83,37.06 v68.27,36.5 | v59.63,36.5 58.36,36.5 IC5.1 | IC8.4 59.64,31.42 59.63,31.29 v59.63,32.05 v67,32.05
  Bottom 0.305: v59.63,32.05 v59.63,36.5 | v68.27,36.5 68.27,33.32 v67,32.05
N$24
  Top 0.305: IC4.6 77.46,35.76 R22.2
N$25  (via drill 0.3)
  Top 0.305: R23.2 v71.56,50.98 v71.57,50.97 | v73.47,36.11 73.09,35.73 71.84,35.73 IC4.3
  Bottom 0.305: v71.57,50.97 71.57,44.75 73.6,42.72 73.6,36.24 v73.47,36.11
N$26
  Top 0.305: IC5.6 63.15,35.14 63.62,34.67 R24.2
N$27  (via drill 0.3)
  Top 0.305: R2.1 41.09,65.93 v41.09,66.84 v41.09,66.85 | 41.09,69.77 v41.09,68.88 S4.2
  Bottom 0.305: v41.09,66.85 v41.09,68.88
N$28
  Top 0.305: IC5.3 56.12,35.14 55.95,34.97 R26.1
N$29
  Top 0.305: S3.2 35.4,66.32 35.76,65.96 35.9,65.86 R33.1
N$30
  Top 0.305: R29.2 36.74,34.97 36.77,34.97 37.03,35.23 42.11,35.23 43.21,34.13 R28.2 43.46,34.13 44.01,33.57 49.6,33.57 51.2,35.18 IC6.6
NRST  (via drill 0.3)
  Top 0.305: IC5.7 v63.57,35.79 | v62.55,27.48 62.48,27.43 49.9,27.43 48.63,26.16 SV2.11 47.28,24.81 40.2,24.81 39.77,25.24 39.77,31.34 39.82,31.39 39.82,31.41 40.94,32.54 R25.1 41.87,32.7 v42.11,32.94 | v45.79,57.96 R32.2
  Bottom 0.305: v62.55,27.48 63.57,28.49 v63.57,35.79 | v42.11,32.94 42.11,36.37 45.15,39.42 45.15,57.32 v45.79,57.96
NRST_IN
  Top 0.305: R28.1 43.3,32.61 40.96,30.27 40.96,28.75 SV2.6
P1.0/MOSI/SDA  (via drill 0.3)
  Top 0.305: U1.12 69,44.27 v70.94,42.34 70.94,41.42 R13.2 | U4.4 74.09,32.57 v73.6,33.07
  Bottom 0.305: v73.6,33.07 70.94,35.73 v70.94,42.34
P1.1/MISO/SCL  (via drill 0.3)
  Top 0.305: U1.11 68.5,43.5 69.54,42.46 v69.54,42.34 69.54,41.42 R14.2 | U4.3 73.32,32.07 v73.22,32.18
  Bottom 0.305: v73.22,32.18 69.54,35.86 v69.54,42.34
P1.2/SPI_CLK  (via drill 0.3)
  Top 0.305: U6.4 65.96,60.52 v66.36,60.12 | v67.25,42.97 67.5,43.22 U1.9
  Bottom 0.305: v66.36,60.12 66.36,43.86 v67.25,42.97
P1.3/SPI_CS  (via drill 0.3)
  Top 0.305: R20.2 64.72,42.47 | 64.72,42.47 65.22,42.97 66.11,42.97 67,43.86 U1.8 | U6.5 62.28,60.52 v61.66,60.5 | 64.71,41.83 v64.71,42.34 64.71,42.46 64.72,42.47
  Bottom 0.305: v61.66,60.5 61.66,45.39 v64.71,42.34
P1.4/TCK  (via drill 0.3)
  Top 0.305: R22.1 v79.05,34.61 | R6.2 50.11,39.29 v50.11,38.02 | v56.33,28.88 56.96,28.24 v75.13,28.24 v78.68,28.24 | U1.22 67.5,50.46 67.51,50.47 67.51,50.59 v67.63,50.72
  Bottom 0.305: v67.63,50.72 69.28,50.72 69.79,50.21 69.79,45.13 72.33,42.59 72.33,35.61 75.13,32.81 v75.13,28.24 | v50.11,38.02 50.11,35.1 v56.33,28.88 | v79.05,34.61 79.05,28.61 v78.68,28.24
P1.5/TDI  (via drill 0.3)
  Top 0.305: U1.21 68,49.94 68.4,50.34 68.4,52.62 66.74,54.28 v64.33,54.28 v54.04,54.28 | R24.1 65.8,35.43 v65.85,35.48 | v53.54,63.42 46.55,63.42 45.66,64.31 45.66,64.33 R1.1
  Bottom 0.305: v65.85,35.48 65.98,35.73 65.98,42.59 64.33,44.24 v64.33,54.28 | v54.04,54.28 54.04,62.91 v53.54,63.42
P1.6/TDO  (via drill 0.3)
  Top 0.305: v49.6,55.04 66.74,55.04 69.03,52.75 69.03,50.21 68.5,49.68 U1.20 | IC6.7 51.28,35.83 v50.87,36.11 | R2.2 41.2,63.44 41.98,62.66 49.47,62.66 | 49.73,62.66 49.47,62.66 | 49.47,62.66 v49.6,62.66 51.63,62.66 53.15,61.14 JMP1.3
  Bottom 0.305: v50.87,36.11 50.87,38.53 49.6,39.8 v49.6,55.04 v49.6,62.66
P1.7/TMS  (via drill 0.3)
  Top 0.305: U1.19 69,49.29 70.17,50.47 70.17,51.86 | 70.17,51.99 70.17,51.86 | 70.17,51.86 70.16,51.88 R23.1 70.17,51.93 70.17,52.37 66.74,55.8 v53.03,55.8 | R33.2 35.87,63.06 37.03,61.89 51.38,61.89 v52.9,60.37
  Bottom 0.305: v52.9,60.37 52.9,55.93 v53.03,55.8
POWER_1V5  (via drill 0.3)
  Top 0.254: TP8.TP 53.79,37.18 C18.2
  Top 0.305: C15.2 IC4.8 74.56,37.06 71.57,40.05 71.03,40.05 R13.1 R14.1 69.57,38.69 68.65,37.64 64.71,37.64 64.46,37.38 64.46,37.24 C16.2 64.09,36.75 63.06,36.75 62.75,36.44 IC5.8 61.82,36.37 v60.77,36.37 59.63,37.51 55.06,37.51 54.68,37.13 54.68,36.37 | IC6.8 54.57,36.48 54.68,36.37 | 54.68,36.37 54.55,36.37 C18.2 | IC8.5 59.78,29.87 60.27,29.89 v60.77,29.89 | 74.47,58.49 74.55,58.49 C3.2 | U6.6 U6.3 64.1,60.02 64.08,59.99 64.08,61.39 64.2,61.51 66.36,61.51 | U4.2 77.68,31.57 C19.2 | 77.67,37.11 77.67,37.89 v77.92,38.15
  Top 0.61: 74.87,58.34 74.47,58.49 IC1.5 74.26,58.49 v74.87,59.1 v73.22,59.1 | S6.3 55.32,71.41 56.84,69.9 v56.84,66.72 | v62.04,61.51 66.36,61.51 68.27,59.61 74.49,59.61 74.87,59.23 C3.2 | 77.67,37.11 C15.2 | 77.68,31.57 77.68,32.45 v77.79,32.56
  Bottom 0.305: v60.77,29.89 v60.77,36.37 | v77.92,38.15 77.92,37.89 77.79,37.77
  Bottom 0.61: v56.84,66.72 v62.04,61.51 | 73.6,59.1 74.11,58.59 | 74.62,58.08 74.11,58.59 | 74.11,58.59 74.75,58.59 74.87,58.72 74.87,46.53 77.92,43.48 v77.92,38.15 | v77.79,32.56 77.79,37.77 77.79,37.89 77.92,38.02 | 73.6,59.1 v74.87,59.1 74.75,59.1 | 73.6,59.1 v73.22,59.1
  pour Top (no thermals): 72.46,59.86 75,59.86 75.25,59.61 75.25,58.21 75.13,58.08 72.46,58.08 70.81,59.74 72.21,59.74 72.33,59.86
POWER_3V3  (via drill 0.3)
  Top 0.254: 74.24,62.53 74.29,62.53 IC2.P$8 | TP7.TP 59.63,59.52
  Top 0.305: R11.1 R10.1 R9.1 | IC2.P$2 IC2.P$7 | IC2.P$1 IC2.P$8 | U6.7 59.63,59.52 59.29,59.52 58.87,59.61 | U7.A 47.03,54.5 v47.06,54.53 | U5.A 46.99,48.37 v47.06,48.31
  Top 0.406: R34.2 48.07,58.91 48.33,58.9
  Top 0.61: v47.44,58.08 R34.2 48.33,58.9 D3.1 50.54,58.9 50.87,59.23 58.49,59.23 58.87,59.61 59,59.74 59,61.01 60.65,62.53 68.37,62.53 IC2.P$1 | v54.04,29.76 58.11,29.76 58.87,29 67.64,29 R11.1 | 74.24,62.53 73.86,62.91 73.86,64.31 72.7,65.46 C5.1 72.7,67.22 73.22,67.74 79.82,67.74 81.35,69.26 81.35,70.69 SV9.1
  Bottom 0.61: v47.44,58.08 47.06,57.7 v47.06,54.53 v47.06,48.31 47.06,36.88 v54.04,29.76
  pour Top (no thermals): 72.71,65.2 72.71,63.42 72.33,63.04 68.14,63.04 67.63,62.53 67.63,62.4 68.27,61.77 75.51,61.77 75.76,62.02 75.76,63.17 72.71,66.21
RF430_RST  (via drill 0.3)
  Top 0.305: v51.76,60.37 47.5,60.37 R34.1
  Top 0.406: R32.1 47.44,60.37 R34.1
  Bottom 0.305: SV9.2 78.97,68.92 77.54,67.48 54.68,67.48 51.76,64.56 v51.76,60.37
RST/NMI  (via drill 0.3)
  Top 0.254: TP10.TP 60.39,39.03
  Top 0.305: U1.10 68,41.53 C11.1 68.07,41.43 R5.1 65.96,41.43 65.6,41.07 65.6,39.42 65.22,39.03 60.39,39.03 v54.3,39.03 52.14,39.03 49.6,36.5 IC6.1 48.69,36.5 46.04,36.5 v45.92,36.62 | S2.P$3 S2.P$4 45.84,56.26 v45.92,56.18 | R26.2 53.99,35.02 v53.79,35.23
  Bottom 0.305: v45.92,56.18 v45.92,36.62 | v53.79,35.23 53.79,36.75 54.3,37.26 v54.3,39.03
TCK  (via drill 0.3)
  Top 0.305: v47.31,32.3 47.57,32.56 58.36,32.56 59.12,33.32 66.49,33.32 69.58,36.41 IC4.2
  Bottom 0.305: SV2.7 43.58,26.16 44.77,27.35 44.77,29.76 v47.31,32.3
TDI  (via drill 0.3)
  Top 0.305: IC5.2 59.2,35.79 59.38,35.61 59.38,34.34 58.11,33.07 45.28,33.07 v45.03,32.81
  Bottom 0.305: v45.03,32.81 43.5,31.29 40.84,31.29 39.69,30.14 39.69,27.39 SV2.3
TDO  (via drill 0.3)
  Top 0.305: SV2.1 35.96,26.16 37.15,27.35 37.15,29.89 v37.79,30.53 | v37.79,30.53 38.55,31.29 R30.2 38.56,31.29 v37.79,30.53 | IC6.3 46.12,35.18 v45.41,34.46
  Bottom 0.305: v45.41,34.46 43.12,32.18 39.44,32.18 v37.79,30.53
TEMP1  (via drill 0.3)
  Top 0.305: R4.2 77.28,50.34 78.33,49.29 SV16.1 | U1.17 75.99,47.52 v76.14,47.67
  Bottom 0.305: v76.14,47.67 77.67,49.19 80.39,49.19 SV16.1
TEMP2
  Top 0.305: U1.18 71.16,48.02 72.59,49.45 75,49.45 75.25,49.19 75.25,48.62 R3.2 76.34,48.49 78.08,46.75 SV16.2
TEST
  Top 0.305: SV2.8 43.54,29.93 44.26,30.65 IC8.2 62.43,30.65 62.66,30.55 R19.2
TMS  (via drill 0.3)
  Top 0.305: IC4.5 74.88,35.11 73.6,33.83 67.76,33.83 66.74,32.81 59.38,32.81 58.11,31.54 v45.15,31.54
  Bottom 0.305: SV2.5 41.04,26.16 42.23,27.35 42.23,30.02 42.61,30.4 44.01,30.4 v45.15,31.54
VDD_2X
  Top 0.305: U1.7 66.5,44.25 65.85,43.61 64.33,43.61 63.44,42.72 63.44,41.58 63.32,41.45 63.46,41.45 C24.2
VDDB  (via drill 0.3)
  Top 0.305: U1.4 61.85,46.52 C12.2
  Top 0.406: C12.2 61.66,45.77 61.28,45.39 60.01,45.39 60,45.39 59.62,45.39 58.62,44.37 56.12,44.37
  Top 0.5: 56.12,44.37 56.08,44.37 SV7.2
  Top 0.61: S6.2 54.66,69.67 55.57,68.75 v55.57,66.47
  Bottom 0.5: 56.08,44.55 56,44.55 SV7.2
  Bottom 0.61: v55.57,66.47 58.36,63.67 58.36,45.64 57.35,44.62 56.08,44.62 56.08,44.55
VDDD
  Top 0.305: U1.24 66.5,49.31 63.93,51.89 C23.1 63.69,53.43 TP2.TP
VDDH
  Top 0.305: U1.23 67,49.7 65.73,50.97 65.73,51.88 C2.1 65.7,53.32 TP1.TP
VDDSW  (via drill 0.3)  (1 unrouted)
  Top 0.254: TP9.TP 58.36,47.16 58.11,47.42
  Top 0.305: S5.1 48.53,67.96 S4.1 43.49,67.96 S3.1 | U1.3 63.58,47.02 62.18,48.42 C13.2 | C13.2
  Top 0.406: JMP1.1 v54.55,64.53 49.63,64.53 48.71,65.45 48.71,67.99 48.7,67.98 S5.1 | C13.2 61.66,47.67 61.41,47.42 58.11,47.42 57.71,47.02 | R5.2 66.57,38.86 65.98,38.27 v52.52,38.27
  Top 0.5: 57.71,47.02 55.96,47.02 SV7.1
  Bottom 0.406: 53.54,47.16 53.54,51.99 55.06,53.51 55.06,63.42 54.55,63.93 v54.55,64.53 | v52.52,38.27 51.76,39.03 51.76,45.25 53.54,47.03 53.54,47.16 | 53.68,47.02 53.54,47.16
  Bottom 0.5: 53.68,47.02 55.93,47.02 SV7.1

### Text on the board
tNames: Supply | S | 0 | 0 | M | 1 | 1 | Battery | 3V3 | PWR | M/S | A1 | A0 | USB For Power Only | U3 | GND | +5V | Reset | +3.3V | ALARM | C | + | * | RF430FRL152HEVM | + | POWER | GND | * | SR66 | 1.55V | Reset | GND | +1.5V | VER:1.01 | GND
